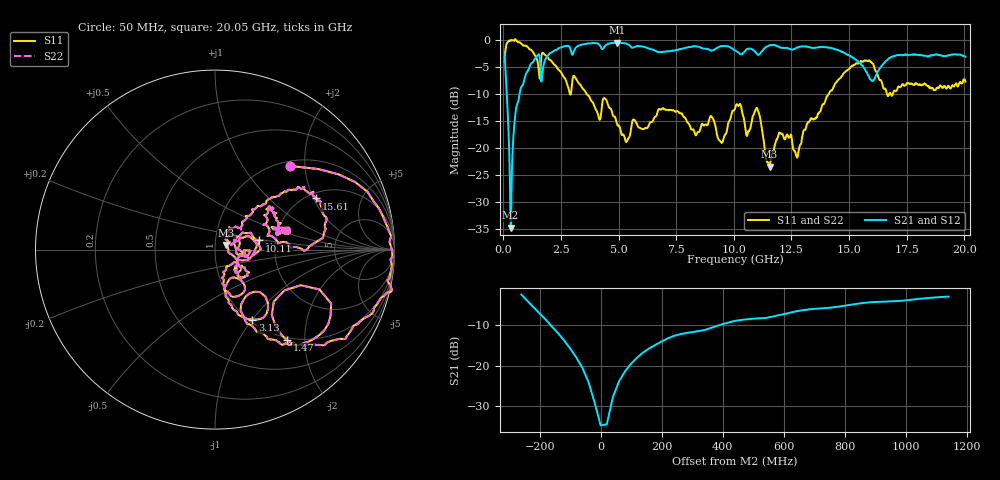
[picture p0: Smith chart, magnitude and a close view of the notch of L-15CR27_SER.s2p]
#	mhz	s	ma	r	50
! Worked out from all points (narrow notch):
!   1001 points, 50 MHz to 20.05 GHz, reference 50 ohm
!   highest |S21| = -0.53 dB at 4.93 GHz (marker M1); lowest = -34.7 dB at 310 MHz (marker M2)
!   notch at M2: 32.8 dB deep, 193 MHz wide at half that depth
!   lowest |S11| = -23.5 dB at 11.55 GHz (marker M3), VSWR 1.14, Z = 56.5 + j2.85 ohm
!   |S11| at or under -10 dB: 3.602 GHz to 14.13 GHz (10.53 GHz wide, 119 % of centre); 16.64 GHz to 16.74 GHz (100.5 MHz wide, 0.602 % of centre); 16.81 GHz to 16.9 GHz (94.49 MHz wide, 0.561 % of centre)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
!   |S22| runs from -23.5 to 0.1 dB; largest |S21 - S12| = 0
!   S11 on the Smith chart (normalised r, x): 50 MHz: 1.09, +1.67; 1.47 GHz: 0.96, -1.64; 3.13 GHz: 1.03, -1.00; 10.11 GHz: 1.64, +0.18; 15.61 GHz: 2.21, +2.08; 20.05 GHz: 2.21, +0.58
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50  0.625 48.2  0.7471 -37.5  0.7471 -37.5  0.625 48.2
310  0.9877 -0.5  0.01836 -19.0  0.01836 -19.0  0.9877 -0.5
650  0.9431 -20.1  0.2734 72.7  0.2734 72.7  0.9431 -20.1
1470  0.6431 -51.5  0.7128 36.2  0.7128 36.2  0.6431 -51.5
1730  0.7516 -39.2  0.5622 43.5  0.5622 43.5  0.7516 -39.2
3130  0.4432 -62.0  0.8388 19.8  0.8388 19.8  0.4432 -62.0
3390  0.3664 -70.6  0.8957 14.7  0.8957 14.7  0.3664 -70.6
4930  0.1674 -74.3  0.9413 -1.6  0.9413 -1.6  0.1674 -74.3
5370  0.1167 -52.4  0.9131 -7.7  0.9131 -7.7  0.1167 -52.4
6730  0.2269 -34.1  0.7661 -11.5  0.7661 -11.5  0.2269 -34.1
9450  0.113 12.7  0.8772 -17.6  0.8772 -17.6  0.113 12.7
10050  0.2305 14.2  0.7957 -25.2  0.7957 -25.2  0.2305 14.2
10110  0.2519 11.7  0.782 -24.7  0.782 -24.7  0.2519 11.7
10610  0.1386 10.4  0.8228 -19.6  0.8228 -19.6  0.1386 10.4
11030  0.2259 1.1  0.7292 -22.7  0.7292 -22.7  0.2259 1.1
11550  0.06699 22.0  0.8842 -21.1  0.8842 -21.1  0.06699 22.0
12750  0.08119 43.7  0.8523 -27.9  0.8523 -27.9  0.08119 43.7
13390  0.1863 40.1  0.8414 -35.4  0.8414 -35.4  0.1863 40.1
15610  0.6295 26.9  0.5649 -55.6  0.5649 -55.6  0.6295 26.9
16170  0.5061 -0.3  0.4687 -26.3  0.4687 -26.3  0.5061 -0.3
16730  0.3098 16.3  0.6723 -25.9  0.6723 -25.9  0.3098 16.3
20050  0.4105 15.3  0.6949 -55.3  0.6949 -55.3  0.4105 15.3
